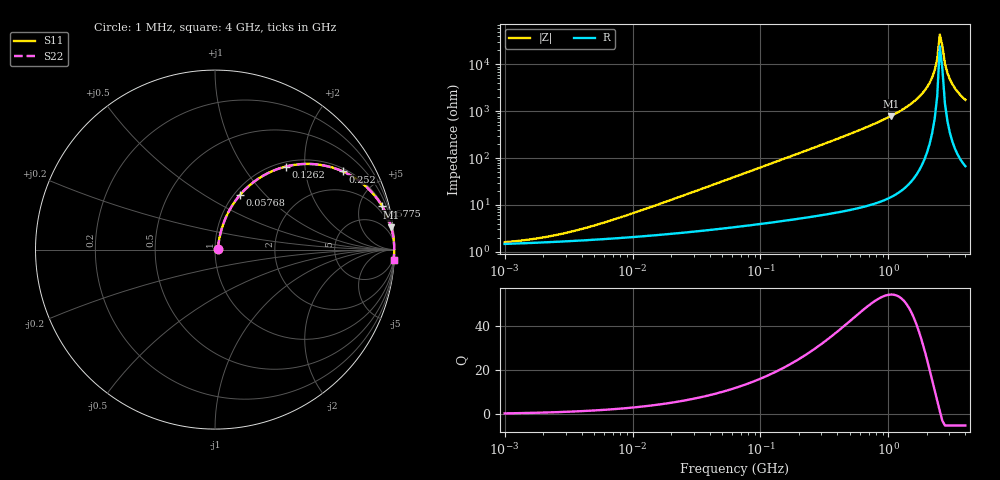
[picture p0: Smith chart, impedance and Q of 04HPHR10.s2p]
# MHz S MA R 50
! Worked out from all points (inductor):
!   181 points, 1 MHz to 4 GHz, reference 50 ohm
!   read as one part in series: L = 100 nH near 10.01 MHz
!   highest Q = 53.9 at 1.051 GHz (marker M1), where L = 120 nH
!   self-resonance near 2.523 GHz
!   S11 on the Smith chart (normalised r, x): 1 MHz: 1.03, +0.01; 57.68 MHz: 1.07, +0.73; 126.2 MHz: 1.09, +1.59; 252 MHz: 1.11, +3.20; 577.5 MHz: 1.17, +7.65; 4 GHz: 2, -35
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1  0.01576 22.8  0.9855 -0.4  0.9855 -0.4  0.01576 22.8
2.09018  0.02031 38.8  0.9842 -0.7  0.9842 -0.7  0.02031 38.8
4.1721  0.03098 54.7  0.9824 -1.5  0.9824 -1.5  0.03098 54.7
16.6226  0.104 71.7  0.9724 -5.8  0.9724 -5.8  0.104 71.7
57.6776  0.3326 65.5  0.9137 -19.3  0.9137 -19.3  0.3326 65.5
63.2456  0.3603 64.1  0.903 -21.0  0.903 -21.0  0.3603 64.1
126.241  0.6073 49.6  0.7627 -37.3  0.7627 -37.3  0.6073 49.6
251.984  0.8349 31.4  0.5219 -56.6  0.5219 -56.6  0.8349 31.4
263.867  0.8463 30.3  0.5047 -57.8  0.5047 -57.8  0.8463 30.3
577.536  0.9623 14.6  0.2516 -74.2  0.2516 -74.2  0.9623 14.6
1051.3  0.9899 7.2  0.1246 -81.8  0.1246 -81.8  0.9899 7.2
1591.59  0.9967 3.5  0.06121 -85.2  0.06121 -85.2  0.9967 3.5
2003.96  0.9983 1.8  0.0308 -85.9  0.0308 -85.9  0.9983 1.8
2197.41  0.9986 1.1  0.01916 -85.2  0.01916 -85.2  0.9986 1.1
2301.03  0.9987 0.8  0.01342 -83.9  0.01342 -83.9  0.9987 0.8
2409.54  0.9987 0.4  0.007729 -80.2  0.007729 -80.2  0.9987 0.4
2523.16  0.9987 0.1  0.0023 -55.8  0.0023 -55.8  0.9987 0.1
2642.15  0.9987 -0.2  0.004035 70.6  0.004035 70.6  0.9987 -0.2
2766.74  0.9986 -0.5  0.009632 81.3  0.009632 81.3  0.9986 -0.5
2897.21  0.9985 -0.9  0.01534 83.8  0.01534 83.8  0.9985 -0.9
3326.7  0.9978 -1.9  0.03277 85.2  0.03277 85.2  0.9978 -1.9
4000  0.9962 -3.3  0.05698 84.5  0.05698 84.5  0.9962 -3.3
